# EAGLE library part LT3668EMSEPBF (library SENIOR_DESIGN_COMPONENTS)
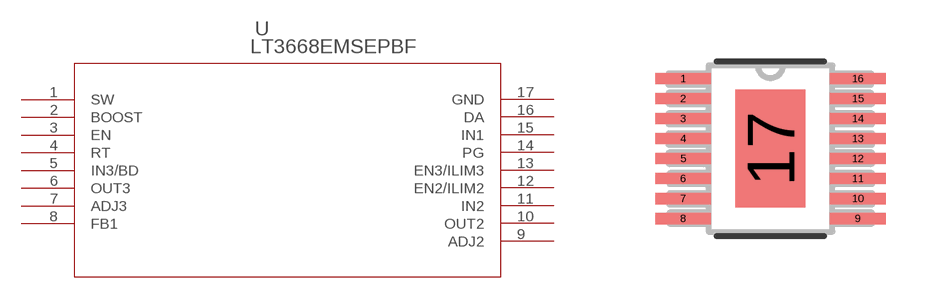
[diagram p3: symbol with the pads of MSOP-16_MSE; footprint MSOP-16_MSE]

Designator prefix U

## LT3668EMSEPBF (DESCRIPTION: LT3668 - 40V 400mA Step-Down Switching Regulator with Dual Fault Protected Tracking LDOs; DIGI-KEY_PART_NUMBER: LT3668EMSE#PBF-ND; DIGI-KEY_PURCHASE_URL: https://www.digikey.com/product-detail/en/linear-technology-analog-devices/LT3668EMSE-PBF/LT3668EMSE-PBF-ND/5030729?utm_source=snapeda&utm_medium=aggregator&utm_campaign=symbol; MF: Linear Technology; MP: LT3668EMSE#PBF; PACKAGE: MSOP-16 Linear Technology)  [MSOP-16_MSE]
1  SW  out
2  BOOST  in
3  EN  pas
4  RT  in
5  IN3/BD  in
6  OUT3  out
7  ADJ3  out
8  FB1  pas
9  ADJ2  out
10  OUT2  out
11  IN2  in
12  EN2/ILIM2  pas
13  EN3/ILIM3  pas
14  PG  out
15  IN1  in
16  DA  pas
17  GND  pwr

## Footprint MSOP-16_MSE (pad centres in mm)
smd 1.397 x 0.279: 1 -2.184,1.751; 2 -2.184,1.251; 3 -2.184,0.751; 4 -2.184,0.25; 5 -2.184,-0.25; 6 -2.184,-0.751; 7 -2.184,-1.251; 8 -2.184,-1.751; 9 2.184,-1.751; 10 2.184,-1.251; 11 2.184,-0.751; 12 2.184,-0.25; 13 2.184,0.25; 14 2.184,0.751; 15 2.184,1.251; 16 2.184,1.751
smd 1.753 x 2.946: 17 0,0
